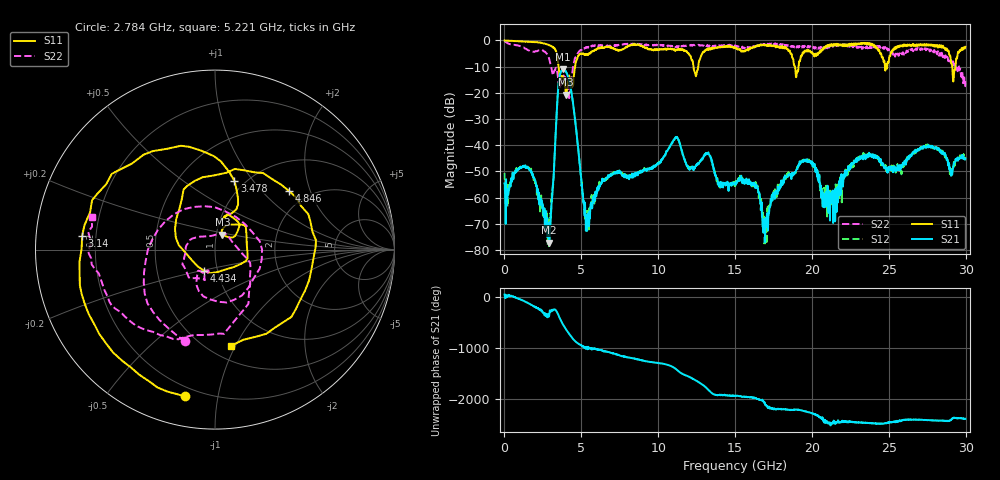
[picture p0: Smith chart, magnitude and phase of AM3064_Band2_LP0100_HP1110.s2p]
# Hz S DB R 50.0
!freq dBS11 angS11 dBS21 angS21 dBS12 angS12 dBS22 angS22
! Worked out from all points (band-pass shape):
!   1600 points, 10 MHz to 29.98 GHz, reference 50 ohm
!   highest |S21| = -11.06 dB at 3.815 GHz (marker M1); lowest = -77.2 dB at 2.915 GHz (marker M2)
!   |S21| within 3 dB of the highest: 3.576 GHz to 4.14 GHz (564.4 MHz wide, 14.6 % of centre)
!   lowest |S11| = -20.7 dB at 4.021 GHz (marker M3), VSWR 1.20, Z = 53.5 + j8.94 ohm
!   |S11| at or under -10 dB: 3.514 GHz to 4.59 GHz (1.076 GHz wide, 26.6 % of centre); 12.29 GHz to 12.6 GHz (312.4 MHz wide, 2.51 % of centre); 18.9 GHz to 19.13 GHz (232 MHz wide, 1.22 % of centre)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
!   |S22| runs from -22.0 to -0.2 dB; largest |S21 - S12| = 0.0074
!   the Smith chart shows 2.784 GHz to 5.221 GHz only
!   S11 on the Smith chart (normalised r, x): 2.784 GHz: 0.15, -0.80; 3.14 GHz: 0.15, +0.05; 3.478 GHz: 0.89, +0.82; 4.434 GHz: 0.86, -0.21; 4.846 GHz: 1.60, +1.45; 5.221 GHz: 0.63, -0.96
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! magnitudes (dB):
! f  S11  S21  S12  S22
! 10 MHz  0.0  -54.6  -50.6  -0.2
! 1.566 GHz  -0.5  -48.9  -48.9  -3.8
! 2.784 GHz  -1.6  -67.7  -68.3  -5.4
! 2.915 GHz  -1.9  -77.2  -77.6  -7.2
! 3.14 GHz  -2.6  -55.8  -56.3  -13.1
! 3.478 GHz  -8.0  -19.7  -19.8  -14.0
! 3.815 GHz  -13.9  -11.1  -11.0  -13.9
! 4.021 GHz  -20.7  -12.1  -12.1  -15.5
! 4.434 GHz  -17.5  -22.8  -22.7  -11.3
! 4.846 GHz  -5.6  -44.1  -44.2  -4.3
! 5.015 GHz  -5.2  -55.6  -53.9  -3.7
! 5.221 GHz  -5.3  -67.0  -67.0  -3.0
! 10 GHz  -3.5  -47.0  -46.9  -1.8
! 11.18 GHz  -3.4  -37.2  -37.0  -2.5
! 15 GHz  -2.7  -54.3  -54.2  -2.0
! 16.35 GHz  -2.3  -55.2  -54.4  -2.4
! 16.92 GHz  -1.8  -69.8  -78.4  -1.5
! 19.99 GHz  -4.5  -46.8  -47.3  -2.3
! 21.23 GHz  -1.8  -62.2  -62.6  -2.5
! 23.1 GHz  -1.4  -44.8  -44.2  -2.5
! 25 GHz  -8.0  -49.2  -48.6  -3.3
! 29.98 GHz  -2.5  -45.2  -45.2  -15.7
